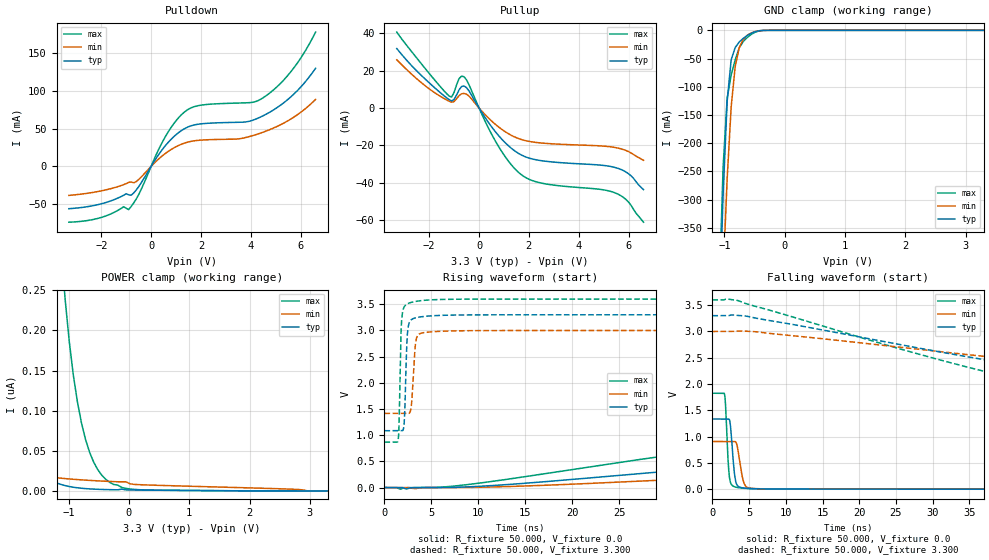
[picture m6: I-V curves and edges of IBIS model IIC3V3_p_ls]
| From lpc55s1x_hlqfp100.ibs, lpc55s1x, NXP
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|   Model IIC3V3_p_ls
[Model] IIC3V3_p_ls
Model_type I/O
Polarity   Non-Inverting
Enable   Active-Low
Vinl =  0.990V
Vinh =  2.310V
Vmeas =  1.650V
Cref =  0.0F
Rref =  100.000
Vref =  0.0V
C_comp   2.367pF   2.322pF   2.392pF
C_comp_pullup   0.514pF   0.423pF   0.587pF
C_comp_pulldown   1.564pF   1.480pF   1.636pF
[Model Spec]
Vinh   2.310V   2.100V   2.520V
Vinl   0.990V   0.900V   1.080V
Vmeas   1.650V   1.500V   1.800V
Vref   0.0V   0.0V   0.0V
Cref   0.0F   0.0F   0.0F
Rref   100.000   100.000   100.000
[Temperature Range]   25.000   0.125k   -40.000
[Voltage Range]   3.300V   3.000V   3.600V
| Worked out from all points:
|   slope of the pulldown table from 0 to 0.495 V, typ, clamps not added: 20.4 ohm
|   slope of the pullup table from 0 to 0.495 V, typ, clamps not added: 49.8 ohm
|   GND clamp passes 1 mA (typ) near -0.43 V on its own axis
|   rising waveform, R_fixture 50.000, V_fixture 0.0: 20-80 % time 64.7ns typ, 78.1ns min, 51.2ns max; typ from 0 V to 1.33 V
|   rising waveform, R_fixture 50.000, V_fixture 3.300: 20-80 % time 240ps typ, 322ps min, 201ps max; typ from 1.08 V to 3.3 V
|   falling waveform, R_fixture 50.000, V_fixture 0.0: 20-80 % time 476ps typ, 652ps min, 377ps max; typ from 1.33 V to 0 V
|   falling waveform, R_fixture 50.000, V_fixture 3.300: 20-80 % time 50.7ns typ, 68.4ns min, 38.4ns max; typ from 3.3 V to 1.09 V
[Pulldown]
|Voltage   I(typ)   I(min)   I(max)
-3.3V     -56mA      -38.4mA    -73.87mA
-2.1V     -50.37mA   -33.07mA   -68.52mA
-1.1V     -38.15mA   -24.11mA   -53.37mA
-900mV    -37.61mA   -21.16mA   -57.18mA
-500mV    -26.92mA   -17.4mA    -37.43mA
500mV     24.51mA    15.34mA    35.14mA
1.2V      47.07mA    29.16mA    67.89mA
1.9V      55.94mA    34.55mA    80.54mA
3.8V      58.93mA    38.31mA    84.23mA
4.5V      67.16mA    45.4mA     91.05mA
5.6V      91.88mA    62.62mA    125.1mA
6.6V      130mA      88.76mA    177.9mA
[Pullup]
|Voltage   I(typ)   I(min)   I(max)
-3.3V     31.81mA    25.76mA    40.62mA
-2.2V     15.96mA    12.29mA    21.78mA
-1.2V     4.465mA    3.611mA    6.352mA
-1.1V     3.737mA    3.067mA    5.829mA
-800mV    9.702mA    6.6mA      15.71mA
-600mV    11.74mA    7.752mA    16.71mA
700mV     -13.46mA   -9.282mA   -18.76mA
1.7V      -25.21mA   -16.93mA   -35.78mA
2.6V      -28.44mA   -18.91mA   -40.52mA
5.5V      -32.06mA   -21.31mA   -45.71mA
6V        -35.26mA   -23.41mA   -50.46mA
6.6V      -43.76mA   -28.06mA   -61.21mA
[GND_clamp]
|Voltage   I(typ)   I(min)   I(max)
-3.3V     -10.05A    -9.18A     -11.33A
-1.089V   -516.5mA   -633.7mA   -475mA
-1.022V   -291.8mA   -436.3mA   -243.2mA
-955mV    -126mA     -264mA     -120.7mA
-888mV    -52.17mA   -135.6mA   -79.11mA
-821mV    -30.43mA   -63.68mA   -52.11mA
-754mV    -20.66mA   -30.68mA   -31.04mA
-687mV    -14.18mA   -15.96mA   -19.64mA
-553mV    -5.013mA   -4.505mA   -7.034mA
-419mV    -652.2uA   -708.2uA   -887.6uA
-285mV    -14.83uA   -32.68uA   -16.3uA
3.3V      0A         0A         0A
[POWER_clamp]
|Voltage   I(typ)   I(min)   I(max)
-3.3V     1.337uA    96.84nA    41.74uA
-2.395V   241.1nA    38.51nA    8.841uA
-2.194V   152.2nA    32.17nA    5.805uA
-1.926V   78.16nA    25.86nA    3.134uA
-1.658V   37.82nA    21.36nA    1.572uA
-1.256V   11.75nA    16.9nA     472.7nA
-1.055V   6.592nA    15.36nA    237.1nA
-921mV    4.605nA    14.51nA    144.1nA
-787mV    3.339nA    13.77nA    84.89nA
-586mV    2.257nA    12.84nA    36.19nA
-318mV    1.588nA    11.83nA    10.67nA
3.3V      0A         0A         0A
[Ramp]
| variable   typ   min   max
dV/dt_r   0.796/64.661n   0.534/78.094n   1.093/51.184n
dV/dt_f   1.328/50.679n   0.947/68.442n   1.640/38.366n
R_load = 50.000
[Rising Waveform]
R_fixture= 50.000
V_fixture= 0.0
V_fixture_min= 0.0
V_fixture_max= 0.0
|time   V(typ)   V(min)   V(max)
0s        11.16nV    74.81nV    32.72nV
1.74ns    77.88uV    92.33nV    -30.99mV
8.05ns    6.84mV     597.9uV    40.21mV
41.16ns   476.1mV    242.5mV    860.7mV
71.46ns   828.1mV    470.5mV    1.45V
84.42ns   980.9mV    550.8mV    1.618V
101.9ns   1.143V     652.9mV    1.726V
123.9ns   1.244V     769mV      1.783V
155.2ns   1.301V     849.9mV    1.812V
200ns     1.326V     890.1mV    1.822V
[Rising Waveform]
R_fixture= 50.000
V_fixture= 3.300
V_fixture_min= 3.000
V_fixture_max= 3.600
|time   V(typ)   V(min)   V(max)
0s        1.085V     1.416V     866.9mV
1.47ns    1.085V     1.416V     919.6mV
1.55ns    1.085V     1.416V     1.176V
1.77ns    1.085V     1.416V     3.001V
1.99ns    1.103V     1.416V     3.4V
2.56ns    3.099V     1.416V     3.52V
2.87ns    3.207V     1.569V     3.538V
3.38ns    3.245V     2.832V     3.557V
4.51ns    3.273V     2.966V     3.58V
200ns     3.3V       3V         3.6V
[Falling Waveform]
R_fixture= 50.000
V_fixture= 0.0
V_fixture_min= 0.0
V_fixture_max= 0.0
|time   V(typ)   V(min)   V(max)
0s        1.334V     906.8mV    1.825V
1.66ns    1.334V     906.8mV    1.806V
1.83ns    1.335V     906.8mV    1.516V
2.22ns    1.335V     906.8mV    372.2mV
2.47ns    1.195V     906.8mV    126.5mV
2.94ns    384.1mV    907.1mV    49.88mV
3.2ns     135.2mV    894.4mV    38.26mV
4.1ns     25.47mV    216.9mV    19.18mV
4.57ns    17.39mV    51.89mV    14mV
200ns     188.6nV    459.6nV    120.2nV
[Falling Waveform]
R_fixture= 50.000
V_fixture= 3.300
V_fixture_min= 3.000
V_fixture_max= 3.600
|time   V(typ)   V(min)   V(max)
0s        3.3V       3V         3.6V
3.32ns    3.308V     3.006V     3.594V
28.42ns   2.676V     2.655V     2.556V
48.9ns    2.199V     2.361V     1.846V
57.16ns   2.033V     2.257V     1.267V
66.11ns   1.791V     2.154V     1.025V
78.16ns   1.371V     2.025V     929.3mV
95.79ns   1.182V     1.724V     887.5mV
127.5ns   1.106V     1.49V      870.5mV
200ns     1.086V     1.421V     867.1mV
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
